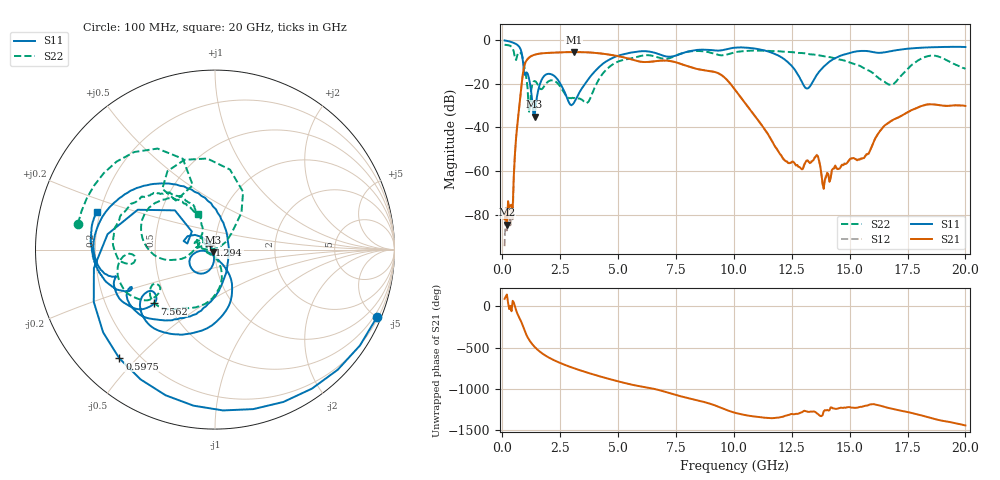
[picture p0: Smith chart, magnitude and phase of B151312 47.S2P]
!  2-Port S-parameters saved by WinCal
! VAR MeasName=S-Parameters (CALIBRATED_DATA) read from VNA (N5244A)
! VAR MeasDate=12/8/2015 5:47:31 PM
! VAR NAME=B151312 47
! VAR FILENAME=B151312 47.S2P
! VAR DATE=12/8/2015 5:47:31 PM
! VAR PHYS_PORTS=1,2
# Hz S DB R 50
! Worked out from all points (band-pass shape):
!   401 points, 100 MHz to 20 GHz, reference 50 ohm
!   highest |S21| = -5.51 dB at 3.085 GHz (marker M1); lowest = -84.6 dB at 199.5 MHz (marker M2)
!   |S21| within 3 dB of the highest: 1.112 GHz to 5.454 GHz (4.342 GHz wide, 132 % of centre)
!   lowest |S11| = -35.2 dB at 1.393 GHz (marker M3), VSWR 1.04, Z = 48.8 - j1.22 ohm
!   |S11| at or under -10 dB: 894.6 MHz to 4.458 GHz (3.564 GHz wide, 133 % of centre); 12.32 GHz to 14.12 GHz (1.799 GHz wide, 13.6 % of centre)
!   |S22| runs from -33.3 to -2.2 dB; largest |S21 - S12| = 0.0018
!   S11 on the Smith chart (normalised r, x): 100 MHz: 0.29, -4.99; 597.5 MHz: 0.13, -0.45; 1.294 GHz: 0.94, +0.05; 7.562 GHz: 0.42, -0.32; 20 GHz: 0.19, +0.15
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1e8  -0.20 -22.6  -82.11 91.0  -94.47 101.5  -2.19 169.3
1.995e8  -0.38 -44.4  -84.65 143.1  -87.25 137.5  -2.28 158.2
3.985e8  -0.94 -87.2  -75.50 -59.1  -78.03 -58.3  -3.03 129.6
5.975e8  -1.86 -131.3  -44.57 -47.8  -44.44 -47.4  -9.13 128.6
9.4575e8  -15.73 142.0  -12.03 79.0  -12.03 79.0  -11.92 54.4
1.14475e9  -17.18 143.6  -8.16 -38.9  -8.16 -38.9  -33.27 26.9
1.294e9  -28.10 138.6  -7.13 -98.0  -7.13 -98.0  -20.37 165.6
1.3935e9  -35.18 -134.2  -6.75 -129.7  -6.75 -129.7  -18.78 148.9
1.64225e9  -19.68 -101.4  -6.19 167.5  -6.19 167.5  -22.43 149.0
2.09e9  -15.60 -146.2  -5.85 88.0  -5.84 88.0  -18.48 165.4
3.085e9  -28.96 -98.5  -5.51 -28.0  -5.51 -28.0  -26.62 -165.7
3.43325e9  -22.23 -66.5  -5.56 -60.7  -5.56 -60.7  -27.30 -151.3
4.72675e9  -8.41 -85.3  -6.86 -167.2  -6.85 -167.2  -11.47 -92.3
6.7665e9  -6.47 -147.5  -9.50 66.5  -9.50 66.4  -8.10 -150.6
7.5625e9  -6.89 -138.4  -10.41 2.4  -10.41 2.4  -6.78 -142.5
1.005e10  -3.50 -175.4  -22.77 151.6  -22.75 151.4  -5.62 -172.5
1.218925e10  -8.86 111.5  -55.03 112.7  -55.15 109.3  -5.36 154.7
1.338325e10  -19.58 -48.1  -55.48 165.0  -55.44 169.4  -6.64 138.3
1.39305e10  -11.74 -89.3  -63.96 -175.5  -64.82 -176.5  -7.54 131.4
1.67165e10  -5.26 -154.9  -37.69 -151.8  -37.57 -152.4  -20.46 154.2
1.8408e10  -3.35 -175.7  -29.49 95.3  -29.46 95.2  -7.32 163.1
2e10  -3.20 162.4  -30.19 -1.7  -30.29 -2.0  -13.24 115.6
